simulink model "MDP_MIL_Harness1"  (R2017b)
settings: Solver=FixedStepDiscrete  StartTime=0.0  StopTime=1  FixedStep=0.01  RelTol=1e-3  EnableMultiTasking=on
undefined symbols (not defined in the file): sigbuilder_block

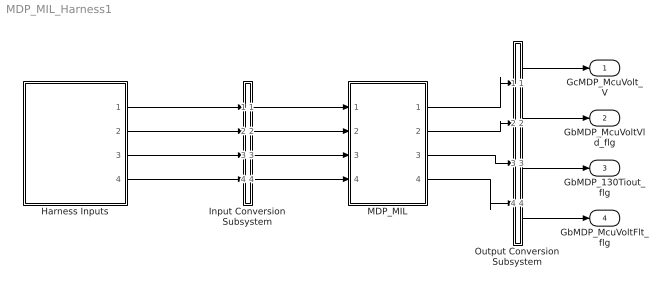
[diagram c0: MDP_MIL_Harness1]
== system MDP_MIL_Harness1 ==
  Harness Inputs : Subsystem  Tag=STV Subsys  LoadFcn=sigbuilder_block('load');  StartFcn=sigbuilder_block('start');  StopFcn=sigbuilder_block('stop');  ClipboardFcn=sigbuilder_block('clipboard');  mask(Sigbuilder block){tuvar=[0:10]}
      mask init:
      | if ~strcmp(get_param(bdroot(gcb),'SimulationStatus'),'stopped'),tuvar = sigbuilder_block('maskInit'); end
  Input Conversion Subsystem : Subsystem  Tag=__SLT_ICS__  Description=Signal spec. and routing
  MDP_MIL : ModelReference  ModelNameDialog=MDP_MIL  SimulationMode=Normal  ModelReferenceVersion='M101C101'
  Output Conversion Subsystem : Subsystem  Tag=__SLT_OCS__  Description=Signal spec. and routing
  GcMDP_McuVolt_V : Outport  OutDataTypeStr=single  PortDimensions=[1]
  GbMDP_McuVoltVld_flg : Outport  Port=2  OutDataTypeStr=boolean  PortDimensions=[1]
  GbMDP_130Tiout_flg : Outport  Port=3  OutDataTypeStr=boolean  PortDimensions=[1]
  GbMDP_McuVoltFlt_flg : Outport  Port=4  OutDataTypeStr=boolean  PortDimensions=[1]
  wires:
  Harness Inputs/1(GcISP_McuVolt_V) -> Input Conversion Subsystem/1(Inport_1)
  Harness Inputs/2(GbISP_130Tiout_flg) -> Input Conversion Subsystem/2(Inport_2)
  Harness Inputs/3(GbVDP_DiagPermit_flg) -> Input Conversion Subsystem/3(Inport_3)
  Harness Inputs/4(GbISP_TF130Tiout_flg) -> Input Conversion Subsystem/4(Inport_4)
  Output Conversion Subsystem/1(Outport_1) -> GcMDP_McuVolt_V/1
  Output Conversion Subsystem/2(Outport_2) -> GbMDP_McuVoltVld_flg/1
  Output Conversion Subsystem/3(Outport_3) -> GbMDP_130Tiout_flg/1
  Output Conversion Subsystem/4(Outport_4) -> GbMDP_McuVoltFlt_flg/1
  Input Conversion Subsystem/1(Outport_1) -> MDP_MIL/1
  Input Conversion Subsystem/2(Outport_2) -> MDP_MIL/2
  Input Conversion Subsystem/3(Outport_3) -> MDP_MIL/3
  Input Conversion Subsystem/4(Outport_4) -> MDP_MIL/4
  MDP_MIL/1 -> Output Conversion Subsystem/1(Inport_1)
  MDP_MIL/2 -> Output Conversion Subsystem/2(Inport_2)
  MDP_MIL/3 -> Output Conversion Subsystem/3(Inport_3)
  MDP_MIL/4 -> Output Conversion Subsystem/4(Inport_4)

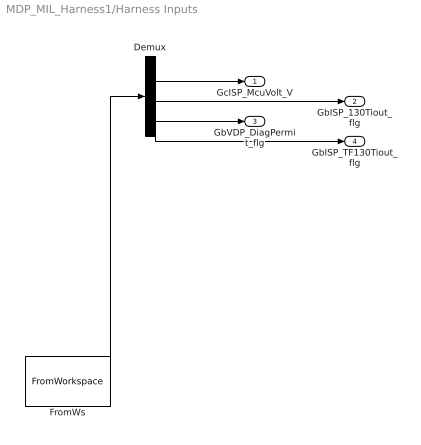
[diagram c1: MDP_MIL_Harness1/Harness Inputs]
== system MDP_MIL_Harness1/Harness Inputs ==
  Demux : Demux  Tag=STV Demux
  FromWs : FromWorkspace  Tag=STV FromWs  VariableName=tuvar  SampleTime=0
  GcISP_McuVolt_V : Outport  Tag=STV Outport
  GbISP_130Tiout_flg : Outport  Tag=STV Outport  Port=2
  GbVDP_DiagPermit_flg : Outport  Tag=STV Outport  Port=3
  GbISP_TF130Tiout_flg : Outport  Tag=STV Outport  Port=4
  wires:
  FromWs/1 -> Demux/1
  Demux/1 -> GcISP_McuVolt_V/1
  Demux/2 -> GbISP_130Tiout_flg/1
  Demux/3 -> GbVDP_DiagPermit_flg/1
  Demux/4 -> GbISP_TF130Tiout_flg/1

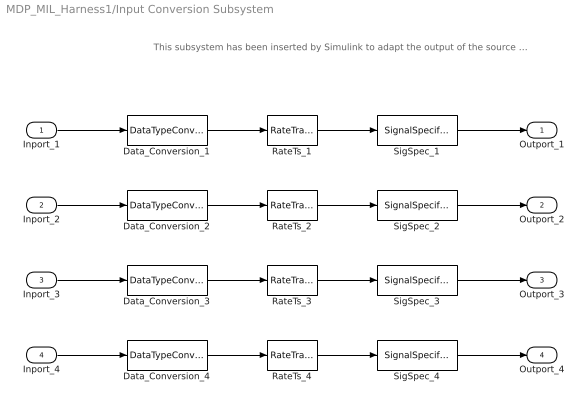
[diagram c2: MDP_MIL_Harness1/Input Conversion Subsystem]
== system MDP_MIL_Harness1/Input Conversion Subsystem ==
  note: This subsystem has been inserted by Simulink to adapt the output of the source blocks to the interface required by the harnessed component. Modifying the contents of this subsystem may result in compilation and simulation failure.
  Inport_1 : Inport
  Inport_2 : Inport  Port=2
  Inport_3 : Inport  Port=3
  Inport_4 : Inport  Port=4
  Data_Conversion_1 : DataTypeConversion  OutDataTypeStr=uint16
  Data_Conversion_2 : DataTypeConversion  OutDataTypeStr=boolean
  Data_Conversion_3 : DataTypeConversion  OutDataTypeStr=boolean
  Data_Conversion_4 : DataTypeConversion  OutDataTypeStr=boolean
  RateTs_{1..4} (4 alike) : RateTransition  OutPortSampleTime=0.01
  SigSpec_1 : SignalSpecification  OutDataTypeStr=uint16  Unit=V  Dimensions=[1]  SampleTime=0.01
  SigSpec_2 : SignalSpecification  OutDataTypeStr=boolean  Unit=flag  Dimensions=[1]  SampleTime=0.01
  SigSpec_3 : SignalSpecification  OutDataTypeStr=boolean  Unit=flg  Dimensions=[1]  SampleTime=0.01
  SigSpec_4 : SignalSpecification  OutDataTypeStr=boolean  Unit=flag  Dimensions=[1]  SampleTime=0.01
  Outport_1 : Outport
  Outport_2 : Outport  Port=2
  Outport_3 : Outport  Port=3
  Outport_4 : Outport  Port=4
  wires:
  SigSpec_1/1 -> Outport_1/1
  RateTs_1/1 -> SigSpec_1/1
  Data_Conversion_1/1 -> RateTs_1/1
  Inport_1/1 -> Data_Conversion_1/1
  SigSpec_2/1 -> Outport_2/1
  RateTs_2/1 -> SigSpec_2/1
  Data_Conversion_2/1 -> RateTs_2/1
  Inport_2/1 -> Data_Conversion_2/1
  SigSpec_3/1 -> Outport_3/1
  RateTs_3/1 -> SigSpec_3/1
  Data_Conversion_3/1 -> RateTs_3/1
  Inport_3/1 -> Data_Conversion_3/1
  SigSpec_4/1 -> Outport_4/1
  RateTs_4/1 -> SigSpec_4/1
  Data_Conversion_4/1 -> RateTs_4/1
  Inport_4/1 -> Data_Conversion_4/1

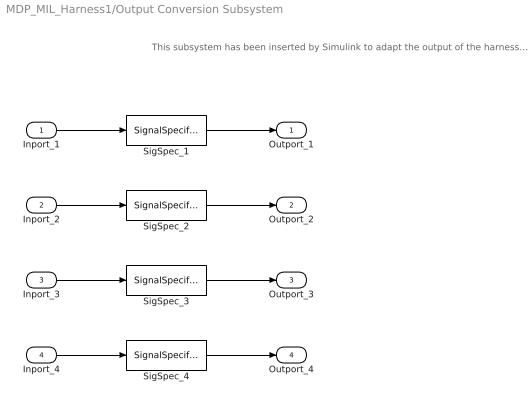
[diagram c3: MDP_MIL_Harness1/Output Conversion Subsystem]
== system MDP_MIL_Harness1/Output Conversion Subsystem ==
  note: This subsystem has been inserted by Simulink to adapt the output of the harnessed component to the interface required by the sink blocks. Modifying the contents of this subsystem may result in compilation and simulation failure.
  Inport_1 : Inport
  Inport_2 : Inport  Port=2
  Inport_3 : Inport  Port=3
  Inport_4 : Inport  Port=4
  SigSpec_1 : SignalSpecification  OutDataTypeStr=single  Unit=V  Dimensions=[1]  SampleTime=0.01
  SigSpec_2 : SignalSpecification  OutDataTypeStr=boolean  Unit=flg  Dimensions=[1]  SampleTime=0.01
  SigSpec_3 : SignalSpecification  OutDataTypeStr=boolean  Unit=flg  Dimensions=[1]  SampleTime=0.01
  SigSpec_4 : SignalSpecification  OutDataTypeStr=boolean  Unit=flg  Dimensions=[1]  SampleTime=0.01
  Outport_1 : Outport
  Outport_2 : Outport  Port=2
  Outport_3 : Outport  Port=3
  Outport_4 : Outport  Port=4
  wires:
  Inport_1/1 -> SigSpec_1/1
  SigSpec_1/1 -> Outport_1/1
  Inport_2/1 -> SigSpec_2/1
  SigSpec_2/1 -> Outport_2/1
  Inport_3/1 -> SigSpec_3/1
  SigSpec_3/1 -> Outport_3/1
  Inport_4/1 -> SigSpec_4/1
  SigSpec_4/1 -> Outport_4/1
